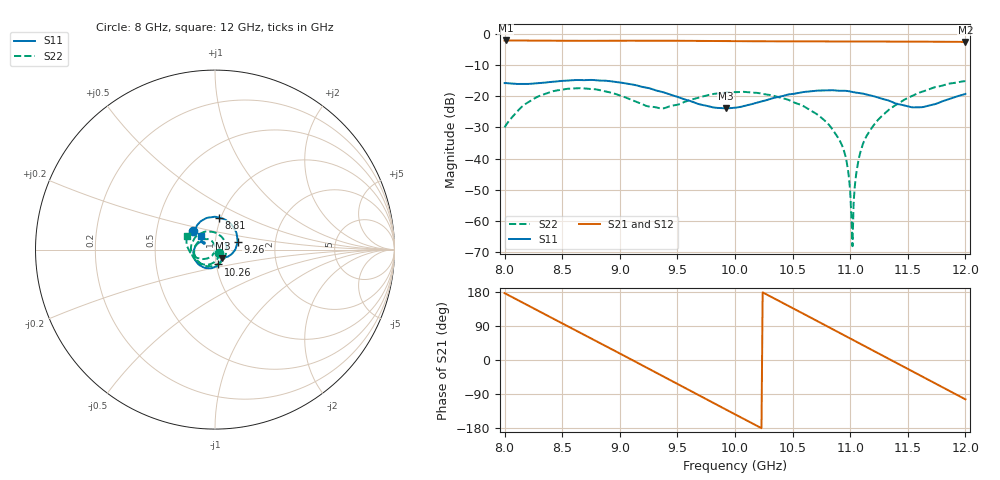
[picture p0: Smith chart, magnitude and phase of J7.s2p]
!Keysight Technologies,N5234A,MY52241180,A.10.60.03
!Date: Tuesday, May 30, 2023 15:25:52
!Correction: S11(Full 2 Port(1,2))
!S21(Full 2 Port(1,2))
!S12(Full 2 Port(1,2))
!S22(Full 2 Port(1,2))
!S2P File: Measurements: S11, S21, S12, S22:
# Hz S  dB  R 50
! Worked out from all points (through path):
!   401 points, 8 GHz to 12 GHz, reference 50 ohm
!   highest |S21| = -2.09 dB at 8.01 GHz (marker M1); lowest = -2.6 dB at 12 GHz (marker M2)
!   group delay of S21, straight-line fit = 445 ps
!   lowest |S11| = -23.9 dB at 9.92 GHz (marker M3), VSWR 1.14, Z = 54.1 - j5.27 ohm
!   |S11| at or under -10 dB: start of sweep to end of sweep
!   |S22| runs from -68.1 to -15.1 dB; largest |S21 - S12| = 0.0015
!   S11 on the Smith chart (normalised r, x): 8 GHz: 0.76, +0.16; 8.81 GHz: 0.98, +0.36; 9.26 GHz: 1.28, +0.12; 10.26 GHz: 1.03, -0.17; 12 GHz: 0.85, +0.13
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8e9  -15.79 139.8  -2.15 176.4  -2.15 176.4  -29.98 -37.9
8.01e9  -15.77 139.7  -2.09 174.9  -2.11 174.9  -29.36 -43.4
8.37e9  -15.52 127.1  -2.17 117.3  -2.18 117.3  -18.99 -136.0
8.67e9  -14.82 99.3  -2.20 69.7  -2.21 69.7  -17.44 168.8
8.81e9  -14.93 82.5  -2.20 47.5  -2.21 47.5  -17.92 142.4
9.04e9  -15.82 51.3  -2.18 10.8  -2.19 10.8  -20.25 93.6
9.26e9  -17.48 19.7  -2.17 -24.5  -2.18 -24.5  -23.33 28.9
9.34e9  -18.39 8.4  -2.17 -37.4  -2.18 -37.4  -23.80 -0.4
9.63e9  -21.76 -28.8  -2.22 -84.1  -2.23 -84.1  -21.03 -90.2
9.92e9  -23.88 -49.4  -2.30 -130.5  -2.31 -130.5  -18.74 -146.4
1e10  -23.69 -54.0  -2.32 -143.3  -2.33 -143.3  -18.68 -159.2
1.026e10  -21.40 -76.8  -2.36 175.3  -2.37 175.2  -19.37 163.8
1.067e10  -18.37 -131.0  -2.39 109.8  -2.40 109.8  -24.86 115.8
1.093e10  -18.25 -167.9  -2.40 68.2  -2.41 68.2  -35.87 87.2
1.097e10  -18.29 -172.9  -2.40 61.8  -2.41 61.8  -41.24 77.8
1.1e10  -18.47 -176.9  -2.40 57.0  -2.41 56.9  -50.62 78.6
1.102e10  -18.64 -179.5  -2.40 53.7  -2.41 53.7  -68.13 -95.0
1.106e10  -18.89 175.3  -2.40 47.3  -2.42 47.3  -43.10 -92.6
1.111e10  -19.15 169.2  -2.41 39.3  -2.42 39.3  -35.40 -101.5
1.134e10  -21.48 148.7  -2.43 2.2  -2.44 2.2  -24.21 -129.0
1.17e10  -22.85 152.4  -2.50 -55.7  -2.51 -55.7  -17.55 -169.6
1.2e10  -19.26 134.9  -2.56 -103.7  -2.57 -103.8  -15.12 153.7
